TYPE "ST_CyclicResponse"
VERSION : 0.1


  STRUCT
   byServiceID : BYTE ;	//Service ID | Service ID related to the request sent by the client
   wDataLength : WORD ;	//Data length | Must be 0x2B in this response (Service ID, Data length, Acknowled
   byAcknowledge : BYTE ;	//Acknowledge | 0x00 if the access was OK or value unequal 0x00 if not | See ackn
   byMessageID : BYTE ;	//Message ID | Message ID related to the request sent by the client
   dwStatusWord : DWORD ;	//Status word | Bit 0 = Manual mode | Bit 1 = Automatic mode | Bit 2 = Homing req
   byComMode : BYTE ;	//Communication mode | 0x00 = Acyclic communication mode | 0x01 = Cyclic communic
   diOffsetForceSensor : DINT ;	//Offset of the force sensor | Unit [N] 1 * 10^-2 (2 decimal places, e.g. 1 = 0,0
   byMotionMode : BYTE ;	//Motion mode (Jog, Move absolute/relative) | 0x00 = Jog | 0x01 = Move absolute |
   diMotionVelocity : DINT ;	//Motion velocity (Jog, Move absolute/relative) | Unit [mm/s] (2 decimal places)
   diMotionPositionDistance : DINT ;	//Motion position/distance (Move absolute/relative) | Unit [mm] (2 decimal places
   wLoadedProgramNumber : WORD ;	//Loaded program number
   byDigitalOutputs : BYTE ;	//Digital outputs (Configurable as output signals in the sequencer of the press p
   diActualPosition : DINT ;	//Actual position | Unit [mm] 1 * 10^-2 (2 decimal places, e.g. 1 = 0,01 mm)
   diActualForce : DINT ;	//Actual force | Unit [N] 1 * 10^-2 (2 decimal places, e.g. 1 = 0,01 N)
   diActualVelocity : DINT ;	//Actual velocity | Unit [mm/s] 1 * 10^-2 (2 decimal places, e.g. 1 = 0,01 mm/s)
   diMaximumPosition : DINT ;	//Maximum position in the press process | Unit [mm] 1 * 10^-2 (2 decimal places,
   diMaximumForce : DINT ;	//Maximum force in the press process | Unit [N] 1 * 10^-2 (2 decimal places, e.g.
   wNOK_Reason : WORD ;	//NOK reason of the press process | More detailed information see online help of
  END_STRUCT ;
END_TYPE

